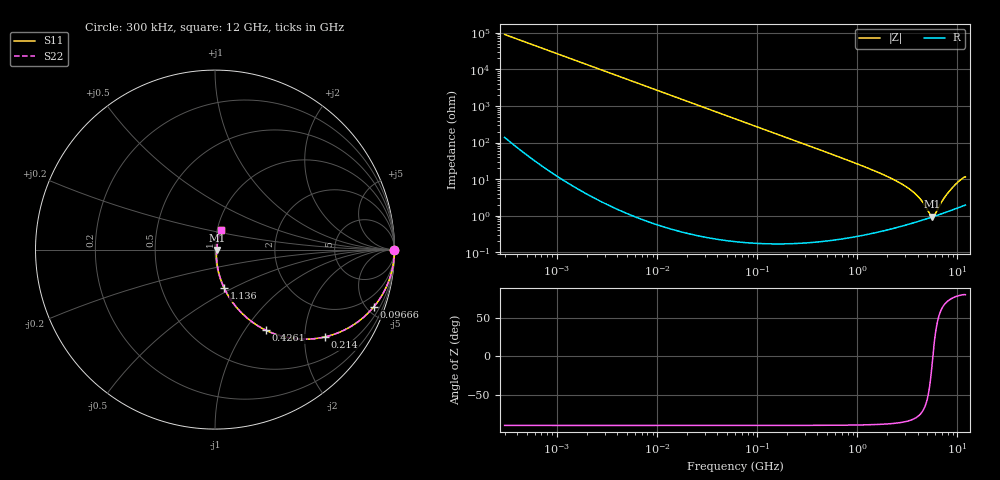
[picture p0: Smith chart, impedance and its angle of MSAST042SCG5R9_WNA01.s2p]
! MSAST042SCG5R9_WNA01  S-PARAMETER MODEL  ( General Type )
! Model Generated by TAIYO YUDEN Corporation (http://www.ty-top.com)
! Version 1.0
! TAIYO YUDEN Control No. 150820
! Copyright(c) 2015 TAIYO YUDEN CO.,LTD. All Rights Reserved.
! Product Description (link to TY-COMPAS)
! https://ds.yuden.co.jp/TYCOMPAS/or/detail?pn=MSAST042SCG5R9BWNA01&u=M
! Products Name : Multilayer Ceramic Capacitors
! Characteristics :
!  Capacitance : 5.9 pF , Rated Voltage : 25V , TCC : CG / C0G
!  Case Size : 0.4 x 0.2 / 0.016 x 0.008 [mm/inch] , Thickness : 0.2 / 0.008 [mm/inch]
!  (Conditions: Temperature = 25 degC , DC Bias Current/Voltage = 0A / 0V)
! External Node Assignments :
!  1  o---| |---o  2
! GND o---------o GND
! Frequency Range : 0.3MHz  -  12000MHz  [ 401 STEP ]
# MHz S RI R 50
! Freq[MHz].  S11 Real  S11 Imag  S21 Real  S21 Imag  S12 Real  S12 Imag  S22 Real  S22 Imag
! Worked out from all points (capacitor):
!   401 points, 300 kHz to 12 GHz, reference 50 ohm
!   read as one part in series: C = 5.91 pF near 316.3 kHz
!   lowest |Z| = 944 mohm at 5.566 GHz (marker M1)
!   series resonance near 5.69 GHz, so ESL is about 130 pH
!   S11 on the Smith chart (normalised r, x): 300 kHz: open; 96.66 MHz: 1.00, -5.57; 214 MHz: 1.00, -2.51; 426.1 MHz: 1.00, -1.26; 1.136 GHz: 1.01, -0.46; 12 GHz: 1.04, +0.23
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0.3  1 -0.00111  2.96e-06 0.00111  2.96e-06 0.00111  1 -0.00111
1.769972  1 -0.00657  4.52e-05 0.00657  4.52e-05 0.00657  1 -0.00657
10.44266  0.9985 -0.0387  0.00151 0.0387  0.00151 0.0387  0.9985 -0.0387
27.82928  0.9894 -0.1022  0.0106 0.1022  0.0106 0.1022  0.9894 -0.1022
60  0.9526 -0.2122  0.0474 0.2122  0.0474 0.2122  0.9526 -0.2122
96.65937  0.8857 -0.3178  0.1143 0.3178  0.1143 0.3178  0.8857 -0.3178
213.9924  0.6123 -0.4866  0.3877 0.4866  0.3877 0.4866  0.6123 -0.4866
353.9943  0.3652 -0.4803  0.6348 0.4803  0.6348 0.4803  0.3652 -0.4803
426.1204  0.2838 -0.4493  0.7162 0.4493  0.7162 0.4493  0.2838 -0.4493
668.5285  0.1378 -0.3418  0.8622 0.3418  0.8622 0.3418  0.1378 -0.3418
1135.593  0.0518 -0.2153  0.9482 0.2153  0.9482 0.2153  0.0518 -0.2153
2088.533  0.0164 -0.1093  0.9836 0.1093  0.9836 0.1093  0.0164 -0.1093
2947.191  0.00977 -0.0658  0.9902 0.0658  0.9902 0.0658  0.00977 -0.0658
3740.715  0.00814 -0.0402  0.9919 0.0402  0.9919 0.0402  0.00814 -0.0402
4385.161  0.00803 -0.0245  0.992 0.0245  0.992 0.0245  0.00803 -0.0245
5278.635  0.00877 -0.00691  0.9912 0.00691  0.9912 0.00691  0.00877 -0.00691
5565.855  0.00914 -0.00196  0.9909 0.00196  0.9909 0.00196  0.00914 -0.00196
6026.253  0.00985 0.00561  0.9901 -0.00561  0.9901 -0.00561  0.00985 0.00561
7254.098  0.0123 0.0257  0.9877 -0.0257  0.9877 -0.0257  0.0123 0.0257
8503.825  0.0159 0.0477  0.9841 -0.0477  0.9841 -0.0477  0.0159 0.0477
10511.28  0.0244 0.0861  0.9756 -0.0861  0.9756 -0.0861  0.0244 0.0861
12000  0.0313 0.1081  0.9687 -0.1081  0.9687 -0.1081  0.0313 0.1081
